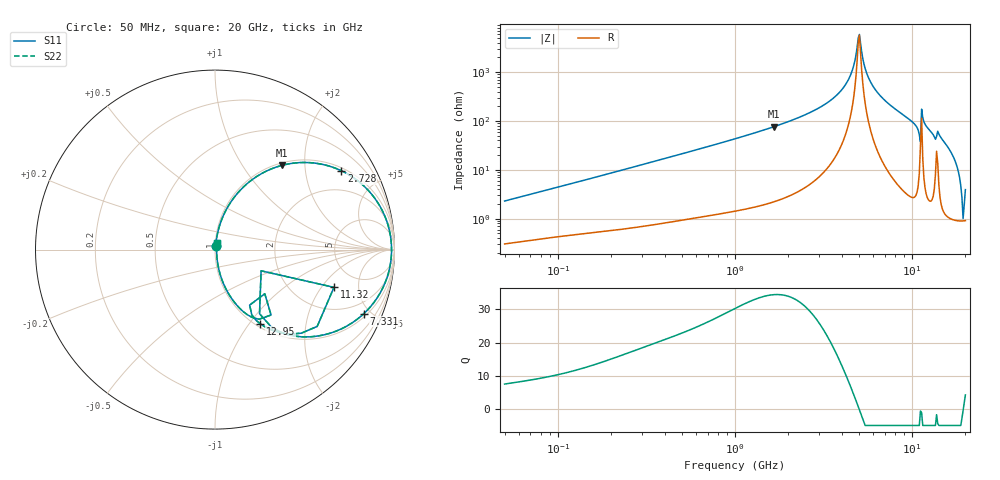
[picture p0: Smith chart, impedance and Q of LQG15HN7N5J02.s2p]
!Murata Part Number: LQG15HN7N5J02
!These Parameters are Measured in Series Mode Connection
!  o--[Z]--o
!Port1  Port2
!  o-------o
!Freq. Start=50[MHz] Stop=20[GHz], 401[Steps]
# Hz S RI R 50
!Freq.(Hz) S11(Real) S11(Imag) S21(Real) S21(Imag) S12(Real) S12(Imag) S22(Real) S22(Imag)
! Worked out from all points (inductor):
!   401 points, 50 MHz to 20 GHz, reference 50 ohm
!   read as one part in series: L = 7.17 nH near 51.52 MHz
!   highest Q = 34.5 at 1.664 GHz (marker M1), where L = 7.34 nH
!   self-resonance near 4.967 GHz
!   S11 on the Smith chart (normalised r, x): 50 MHz: 1.01, +0.05; 2.728 GHz: 1.11, +3.13; 7.331 GHz: 1.18, -4.57; 11.32 GHz: 3.27, -2.66; 12.95 GHz: 1.05, -1.13; 20 GHz: 1.02, +0.08
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5e7  0.00355 0.0227  0.9964 -0.0227  0.9964 -0.0227  0.00355 0.0227
1.364002e8  0.00831 0.0586  0.9917 -0.0586  0.9917 -0.0586  0.00831 0.0586
3.721004e8  0.0316 0.1521  0.9684 -0.1521  0.9684 -0.1521  0.0316 0.1521
1e9  0.165 0.3551  0.835 -0.3551  0.835 -0.3551  0.165 0.3551
1.664083e9  0.3741 0.4696  0.6259 -0.4696  0.6259 -0.4696  0.3741 0.4696
2.728004e9  0.7039 0.4394  0.2961 -0.4394  0.2961 -0.4394  0.7039 0.4394
4.149438e9  0.9486 0.1806  0.0514 -0.1806  0.0514 -0.1806  0.9486 0.1806
4.539627e9  0.9736 0.0985  0.0264 -0.0985  0.0264 -0.0985  0.9736 0.0985
5.041459e9  0.9838 -0.00417  0.0162 0.00417  0.0162 0.00417  0.9838 -0.00417
5.769027e9  0.9637 -0.1397  0.0363 0.1397  0.0363 0.1397  0.9637 -0.1397
7.331367e9  0.8301 -0.3561  0.1699 0.3561  0.1699 0.3561  0.8301 -0.3561
7.442007e9  0.8177 -0.3674  0.1823 0.3674  0.1823 0.3674  0.8177 -0.3674
9.892087e9  0.4995 -0.4864  0.5005 0.4864  0.5005 0.4864  0.4995 -0.4864
1.082228e10  0.3118 -0.429  0.6882 0.429  0.6882 0.429  0.3118 -0.429
1.131968e10  0.6628 -0.2104  0.3372 0.2104  0.3372 0.2104  0.6628 -0.2104
1.183995e10  0.4262 -0.4705  0.5738 0.4705  0.5738 0.4705  0.4262 -0.4705
1.295331e10  0.2517 -0.4131  0.7483 0.4131  0.7483 0.4131  0.2517 -0.4131
1.438523e10  0.2051 -0.377  0.7949 0.377  0.7949 0.377  0.2051 -0.377
1.670968e10  0.0538 -0.2043  0.9462 0.2043  0.9462 0.2043  0.0538 -0.2043
1.800918e10  0.0207 -0.1071  0.9793 0.1071  0.9793 0.1071  0.0207 -0.1071
1.912117e10  0.00956 -0.0252  0.9904 0.0252  0.9904 0.0252  0.00956 -0.0252
2e10  0.0105 0.0375  0.9895 -0.0375  0.9895 -0.0375  0.0105 0.0375
